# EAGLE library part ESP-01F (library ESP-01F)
802.11b/g/n Wi-Fi SOC module Check availability
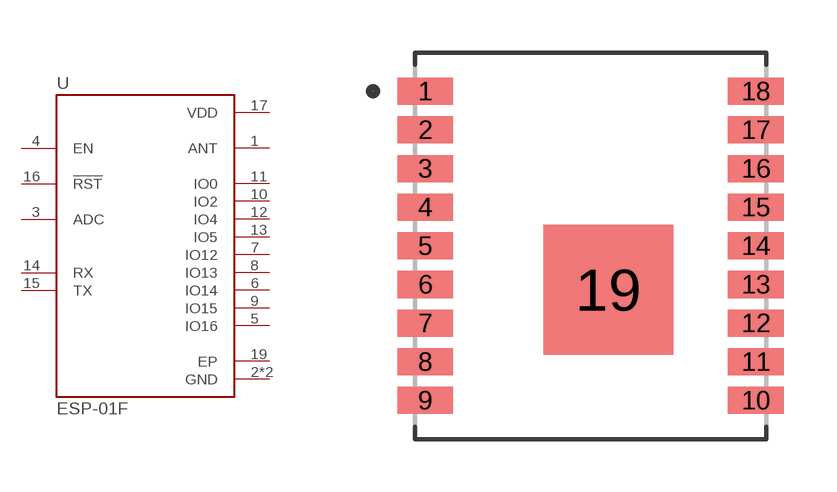
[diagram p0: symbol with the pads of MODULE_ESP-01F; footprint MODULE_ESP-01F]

Designator prefix U

## ESP-01F (Availability: Not in stock; Description: 802.11b/g/n Wi-Fi SOC module; MF: AI-Thinker; MP: ESP-01F; Package: None; Price: None)  [MODULE_ESP-01F]
1  ANT
2  GND  pwr
3  ADC  in
4  EN  in
5  IO16
6  IO14
7  IO12
8  IO13
9  IO15
10  IO2
11  IO0
12  IO4
13  IO5
14  RX  in
15  TX  out
16  !RST  in
17  VDD  pwr
18  GND  pwr
19  EP  pas

## Footprint MODULE_ESP-01F (pad centres in mm)
smd 1.59 x 0.77: 1 -4.71,4.4; 2 -4.71,3.3; 3 -4.71,2.2; 4 -4.71,1.1; 5 -4.71,0; 6 -4.71,-1.1; 7 -4.71,-2.2; 8 -4.71,-3.3; 9 -4.71,-4.4; 10 4.71,-4.4; 11 4.71,-3.3; 12 4.71,-2.2; 13 4.71,-1.1; 14 4.71,0; 15 4.71,1.1; 16 4.71,2.2; 17 4.71,3.3; 18 4.71,4.4
smd 3.7 x 3.7: 19 0.5,-1.25

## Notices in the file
This work is licensed under a Creative Commons Attribution-ShareAlike 4.0 International License (CC BY-SA) with Design Exception 1.0
